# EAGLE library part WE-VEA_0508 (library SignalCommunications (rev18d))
WE-VEA ESD Suppressor-Array Characteristics Fast response time (1 ns) Low signal insertion loss No leakage current Low clamping voltage Almost no energy consumption in stand-by mode Excellent absorption for ESD-impulses Operating temperature: –40 ºC to +85 ºC Applications Protection of data lines Protection of bus systems Protection of video transmission lines Protection of semiconductors ESD protection in accordance with EN 61000-4-2 Details see: http://katalog.we-online.de/en/pbs/WE-VEA? Updated by Dan Xu 2014-07-11 2014 (C) Wurth Elektronik
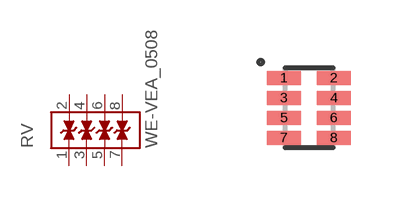
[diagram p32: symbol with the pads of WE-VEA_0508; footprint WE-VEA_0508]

Designator prefix RV

## WE-VEA_0508_82380050100  [WE-VEA_0508]
1  1  pas
2  8  pas
3  2  pas
4  7  pas
5  3  pas
6  6  pas
7  4  pas
8  5  pas

## Footprint WE-VEA_0508 (pad centres in mm)
WESURGE ESD Suppressor-Array WE-VEA
smd 0.85 x 0.35: 1 -0.625,0.75; 2 0.625,0.75; 3 -0.625,0.25; 4 0.625,0.25; 5 -0.625,-0.25; 6 0.625,-0.25; 7 -0.625,-0.75; 8 0.625,-0.75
